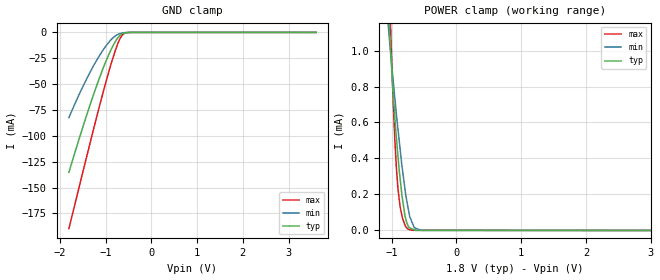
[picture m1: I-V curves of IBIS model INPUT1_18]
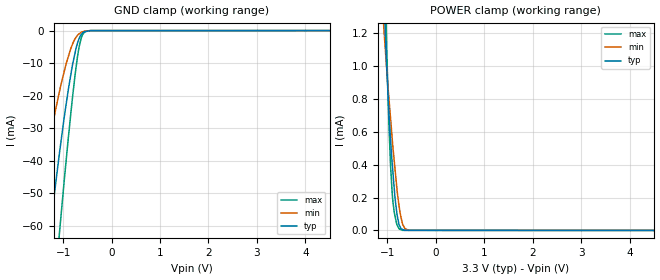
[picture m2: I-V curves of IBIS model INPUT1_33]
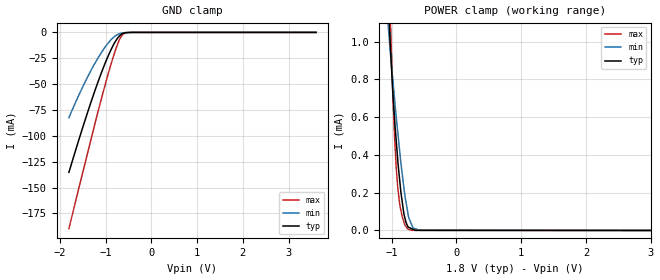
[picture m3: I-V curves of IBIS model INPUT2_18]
|Texas Instruments Incorporated
|Low Distortion Digital-to-Analog Converter for Seismic Monitoring
| Marketing part#   Digital Voltage Range   Package-type   #pins
|DAC1280IPW   1.65 to 3.6   TSSOP   16
|DAC1280IPWR   1.65 to 3.6   TSSOP   16
[IBIS Ver]   3.2
[File name]   dac1280.ibs
[File Rev]   1.0
[Date]   10/06/2010
[Source]   Texas Instruments Incorporated.
   Analog-eLab, HPA
   12500 TI Blvd
   Dallas, TX -75243
   For Support e-mail: elab_ibis@list.ti.com
[Notes]   Revision History:
   1.0: 10/06/2010
   - Initial version of the model
   - Initial Model generated from simulations in TISPICED
   - Model names with a trailing _18 contains the model for
   1.8V (1.65V and 1.98V).
   _ Model names with trailing _33 contains
   the model for 3.3V (3.0V and 3.6V) operation.
   - Model not matched to measurements
   - C_comp although listed in numerical order of value are
   obtained from varying PVT conditions. For PVT conditions
   for each specific value refer the buffer description under
   respective [Model]. IBIS model user is responsible for using
   appropriate C_comp to simulate for Signal Integrity.
[Disclaimer]
 This product is designed as an aid for customers of Texas Instruments.
 No warranties, either expressed or implied, with respect to this third
 party software (if any) or with respect to its fitness for any
 particular purpose is claimed by Texas Instruments or the author. The
 software (if any) is provided solely on an "as is" basis. The entire
 risk as to its quality and performance is with the customer
[Copyright] (C) Copyright 2009 Texas Instruments Incorporated.
   All rights reserved.
|   ADSxxxx
[Component]   DAC1280
[Manufacturer] TI
[Package]   | 16 TSSOP - PW package
| variable   typ   min   max
R_pkg  5.68555E-02   2.62900E-02   7.97800E-02
L_pkg  2.17370E+00nH 1.39515E+00nH 3.11425E+00nH
C_pkg  3.02345E-01pF 2.47820E-01pF 3.60470E-01pF
|-------------------------PIN------------------------------------------------
[Pin] signal_name  model_name  R_pin  L_pin C_pin
1   CLK   INPUT1   0.06846  2.87680nH  0.34612pF
2   TDATA   INPUT1   0.06088  1.84077nH  0.25943pF
3   SYNC   INPUT1   0.04853  1.59862nH  0.24782pF
4   DGND   GND   0.02436  1.32007nH  0.27215pF
5   DVDD   POWER   0.02447  1.32337nH  0.27328pF
6   GAIN0   INPUT1   0.05274  1.68343nH  0.25385pF
7   GAIN1   INPUT1   0.06868  2.00258nH  0.27020pF
8   GAIN2   INPUT1   0.07978  3.11425nH  0.36032pF
9   VREF   TERM   0.07830  3.08425nH  0.36047pF
10   RREF   TERM   0.03457  1.70225nH  0.30454pF
11   AVSS   POWER   0.02040  1.42921nH  0.31877pF
12   AVDD   POWER   0.02701  1.40290nH  0.28306pF
13   NC   NC   0.00151  0.89617nH  0.19593pF
14   IOUTN   TERM   0.02629  1.39515nH  0.27970pF
15   IOUTP   TERM   0.03242  1.60905nH  0.29286pF
16   _PWDN   INPUT2   0.07476  3.00360nH  0.35048pF
|   Model Selectors
[Model Selector]  INPUT1
INPUT1_18   1.8V digital input
INPUT1_33   3.3V digital input
|NOTES   Model INPUT1 split into two Models INPUT1_18 and INPUT1_33
|   to accomodate vast voltage range of 1.65V to 3.6V
|   INPUT1_18 operates in voltage range of 1.65 - 1.8 - 1.98
|   INPUT1_33 operates in voltage range of 3.0 - 3.3 - 3.6
|   The max pin frequency for Model INPUT1 is 4MHz.Also the
|   voltage range and frequency is referenced with datasheet.
[Model Selector]  INPUT2
INPUT2_18   1.8V digital input
INPUT2_33   3.3V digital input
|NOTES   Model INPUT2 split into two Models INPUT2_18 and INPUT2_33
|   to accomodate vast voltage range of 1.65V to 3.6V
|   INPUT2_18 operates in voltage range of 1.65 - 1.8 - 1.98
|   INPUT2_33 operates in voltage range of 3.0 - 3.3 - 3.6
|   The max pin frequency for Model INPUT2 is 100kHz.Also the
|   voltage range and frequency is referenced with datasheet.
[Model Selector]  TERM
TERM_18   1.8V digital input
TERM_33   3.3V digital input
|   TERM_18 Model
[Model] TERM_18
Model_type Terminator
C_comp   0   0   0
| variable   typ   min   max
[Voltage Range]   1.8V   1.65V   1.98V
[POWER Clamp Reference]  1.8V   1.65V   1.98V
[GND Clamp Reference]   0.0V   0.0V   0.0V
|Operating Temperature
[Temperature Range]   27   85   -40
|   TERM_33 Model
[Model] TERM_33
Model_type Terminator
C_comp   0   0   0
| variable   typ   min   max
[Voltage Range]   3.3V   3.0V   3.3V
[POWER Clamp Reference]  3.3V   3.0V   3.3V
[GND Clamp Reference]   0.0V   0.0V   0.0V
|Operating Temperature
[Temperature Range]   27   85   -40
| Models and submodels in the file (6): INPUT1_18 (Input), INPUT1_33 (Input), INPUT2_18 (Input), INPUT2_33 (Input), TERM_18 (Terminator), TERM_33 (Terminator)
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|NOTES   Model DIN split into two Models TERM_18 and TERM_33
|   to accomodate vast voltage range of 1.65V to 3.6V
|   TERM_18 operates in voltage range of 1.65 - 1.8 - 1.98
|   TERM_33 operates in voltage range of 3.0 - 3.3 - 3.6
|   The max pin frequency for Model TERM is 4MHz.Also the
|   voltage range and frequency is referenced with datasheet.
|   INPUT1_18   1.8V digital input Model
[Model]   INPUT1_18
Model_type   Input
| Signals : CLK(1), TDATA(2), SYNC(3), GAIN0(6), GAIN1(7), GAIN2(8)
Vinl = 0.36
Vinh = 1.44
|   typ   min   max
|   (nom PVT)   (Fast PVT)   (slow PVT)
C_comp   2.7751000e-12   2.0530600e-12  3.5150200e-12
| Where   nom PVT is  Nominal Process, 1.8V, 27C
|   Fast PVT is Strong Process, 1.98V, -40C
|   Slow PVT is Weak Process, 1.65V, 85C
[Voltage Range]   1.8   1.65   1.98
[Temperature Range]   27   85   -40
[Power Clamp Reference]   1.8   1.65   1.98
[GND Clamp Reference]   0   0   0
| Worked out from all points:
|   GND clamp passes 1 mA (typ) near -0.62 V on its own axis
|   POWER clamp passes 1 mA (typ) near -1.02 V on its own axis
[GND Clamp]
|   Voltage   I(typ)   I(min)   I(max)
-1.8V     -135.3mA   -82.39mA   -189.7mA
-1.616V   -108.7mA   -63.88mA   -156.7mA
-1.378V   -75.55mA   -41.97mA   -114.3mA
-1.229V   -56.07mA   -29.7mA    -88.04mA
-1.062V   -35.76mA   -17.62mA   -59.52mA
-932.8mV  -21.85mA   -9.858mA   -38.83mA
-792.5mV  -9.397mA   -3.625mA   -18.42mA
-708.8mV  -4.106mA   -1.549mA   -8.381mA
-674.5mV  -2.592mA   -997.2uA   -5.258mA
-610.8mV  -857.3uA   -415.8uA   -1.619mA
-439.3mV  -12.68uA   -10.92uA   -11.24uA
3.6V      0A         0A         0A
[POWER Clamp]
|   Voltage   I(typ)   I(min)   I(max)
-1.8V     10.49mA    8.185mA    13.21mA
-1.048V   1.242mA    1.117mA    1.514mA
-1.034V   1.136mA    1.059mA    1.339mA
-1.014V   993.3uA    976uA      1.112mA
-979.5mV  772.8uA    843.3uA    744.8uA
-950.6mV  624.8uA    734.8uA    500.3uA
-901.8mV  409.1uA    560.5uA    229.9uA
-841.6mV  195.7uA    359.8uA    83.58uA
-753.3mV  31.53uA    139.2uA    8.181uA
-650.6mV  3.533uA    15.48uA    979.2nA
-544.7mV  636.7nA    629.2nA    954.8nA
3.6V      0A         0A         0A
|   INPUT1_33   3.3V digital input Model
[Model]   INPUT1_33
Model_type   Input
| Signals : CLK(1), TDATA(2), SYNC(3), GAIN0(6), GAIN1(7), GAIN2(8)
Vinl = 0.66
Vinh = 2.34
|   typ   min   max
|   (nom PVT)   (Fast PVT)   (slow PVT)
C_comp   2.5280580e-12   1.8984050e-12   3.2362170e-12
| Where   nom PVT is  Nominal Process, 3.3V, 27C
|   Fast PVT is Strong Process, 3.6V, -40C
|   Slow PVT is Weak Process, 3.0V, 85C
[Voltage Range]   3.3   3   3.6
[Temperature Range]   27   85   -40
[Power Clamp Reference]   3.3   3   3.6
[GND Clamp Reference]   0   0   0
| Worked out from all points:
|   GND clamp passes 1 mA (typ) near -0.62 V on its own axis
|   POWER clamp passes 1 mA (typ) near -1.01 V on its own axis
[GND Clamp]
|   Voltage   I(typ)   I(min)   I(max)
-3.3V     -365.5mA   -259mA     -460.3mA
-1.595V   -105.6mA   -61.89mA   -152.8mA
-1.294V   -64.37mA   -34.83mA   -99.33mA
-1.194V   -51.58mA   -27.04mA   -81.93mA
-1.087V   -38.73mA   -19.4mA    -63.81mA
-1.063V   -36mA      -17.71mA   -59.7mA
-891.5mV  -17.81mA   -7.842mA   -32.5mA
-809.7mV  -10.66mA   -4.242mA   -20.73mA
-702.2mV  -3.735mA   -1.418mA   -7.727mA
-622.9mV  -1.055mA   -471.7uA   -2.094mA
-433.7mV  -11.67uA   -12.53uA   -9.215uA
6.6V      0A         0A         0A
[POWER Clamp]
|   Voltage   I(typ)   I(min)   I(max)
-3.3V     30.98mA    25.71mA    38.1mA
-1.075V   1.482mA    1.236mA    1.87mA
-1.052V   1.278mA    1.14mA     1.565mA
-1.021V   1.041mA    1.011mA    1.195mA
-968.1mV  712uA      803.3uA    642.7uA
-937mV    564.5uA    690.4uA    408.2uA
-901.9mV  413.5uA    562.8uA    230.7uA
-832.6mV  171.5uA    343uA      73.63uA
-757.9mV  33.79uA    147.5uA    9.536uA
-684.2mV  6.013uA    36.88uA    781.9nA
-558.4mV  878.6nA    962nA      768.4nA
6.6V      0A         0A         0A
|   INPUT2_18   1.8V digital input Model
[Model]   INPUT2_18
Model_type   Input
|  Signals : _PWDN(16)
Vinl = 0.36
Vinh = 1.44
|   typ   min   max
|   (nom PVT)   (Fast PVT)   (slow PVT)
C_comp   2.7273880e-12   1.9750560e-12   3.5097250e-12
| Where   nom PVT is  Nominal Process, 1.8V, 27C
|   Fast PVT is Strong Process, 1.98V, -40C
|   Slow PVT is Weak Process, 1.65V, 85C
[Voltage Range]   1.8   1.65   1.98
[Temperature Range]   27   85   -40
[Power Clamp Reference]   1.8   1.65   1.98
[GND Clamp Reference]   0   0   0
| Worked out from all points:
|   GND clamp passes 1 mA (typ) near -0.62 V on its own axis
|   POWER clamp passes 1 mA (typ) near -1.02 V on its own axis
[GND Clamp]
|   Voltage   I(typ)   I(min)   I(max)
-1.8V     -135.3mA   -82.39mA   -189.7mA
-1.616V   -108.7mA   -63.88mA   -156.7mA
-1.379V   -75.57mA   -41.98mA   -114.3mA
-1.23V    -56.14mA   -29.74mA   -88.13mA
-1.062V   -35.84mA   -17.66mA   -59.61mA
-932.5mV  -21.81mA   -9.837mA   -38.75mA
-792.7mV  -9.399mA   -3.624mA   -18.42mA
-709mV    -4.1mA     -1.551mA   -8.389mA
-674.7mV  -2.584mA   -992.8uA   -5.262mA
-611mV    -858.6uA   -415.2uA   -1.62mA
-440mV    -12.33uA   -13.17uA   -11.39uA
3.6V      0A         0A         0A
[POWER Clamp]
|   Voltage   I(typ)   I(min)   I(max)
-1.8V     10.43mA    8.127mA    13.16mA
-1.051V   1.214mA    1.076mA    1.506mA
-1.037V   1.102mA    1.014mA    1.323mA
-1.017V   953.2uA    928.3uA    1.088mA
-954.5mV  588uA      692.9uA    491.3uA
-907.1mV  378.3uA    524.9uA    231.9uA
-870.3mV  246.8uA    400.7uA    128.8uA
-813.8mV  94.97uA    234.6uA    48.61uA
-753.5mV  23.33uA    100.5uA    8.199uA
-670.2mV  5.85uA     13.5uA     989.2nA
-565.3mV  691.1nA    573.6nA    964.8nA
3.6V      0A         0A         0A
